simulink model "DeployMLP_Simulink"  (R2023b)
settings: Solver=VariableStepAuto  StartTime=0.0  StopTime=1  RelTol=1e-3
undefined symbols (not defined in the file or in its folder): test_array_sim

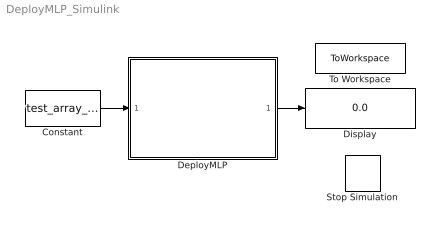
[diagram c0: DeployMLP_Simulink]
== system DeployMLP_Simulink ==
  Constant : Constant  Value=test_array_sim
  DeployMLP : Subsystem  ReferencedSubsystem=DeployMLP  W_conc=W_conc  b_conc=b_conc  scale=scale  decoding_matrix=decoding_matrix
  Display : Display
  Stop Simulation : Stop
  To Workspace : ToWorkspace  VariableName=Y  SampleTime=-1
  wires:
  Constant/1 -> DeployMLP/1
  DeployMLP/1 -> Display/1
